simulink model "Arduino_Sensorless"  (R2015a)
settings: Solver=ode45  StartTime=0.0  StopTime=10.0  RelTol=1e-3
libraries: dspsigops x12, arduinolib x11, simulink x7

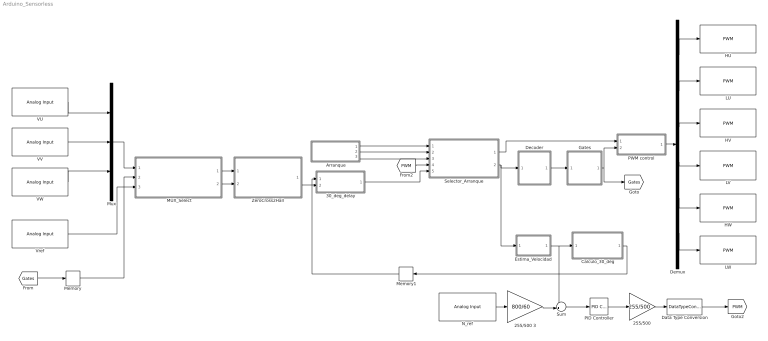
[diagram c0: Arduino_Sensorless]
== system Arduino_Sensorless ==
  " MUX_Select" : Subsystem
  "255/500 " : Gain  Gain=255/500
  255/500 3 : Gain  Gain=800/60
  30_deg_delay : Subsystem
  Arranque : Subsystem
  Calculo_30_deg : Subsystem
  Data Type Conversion : DataTypeConversion  OutDataTypeStr=int16  RndMeth=Round
  Decoder : Subsystem
  Demux : Demux  Outputs=6
  Estima_Velocidad : Subsystem
  Gates : Subsystem
  HU : arduinolib/PWM  pinNumber=3  blockPlatform=arduino
  HV : arduinolib/PWM  pinNumber=6  blockPlatform=arduino
  HW : arduinolib/PWM  pinNumber=10  blockPlatform=arduino
  LU : arduinolib/PWM  pinNumber=5  blockPlatform=arduino
  LV : arduinolib/PWM  pinNumber=9  blockPlatform=arduino
  LW : arduinolib/PWM  pinNumber=11  blockPlatform=arduino
  Memory : Memory
  Memory1 : Memory
  Mux : Mux  Inputs=3
  N_ref : arduinolib/Analog Input  pinNumber=0  sampleTime=1  blockPlatform=arduino
  PID Controller : simulink/Continuous/PID Controller  Controller=PID  TimeDomain=Continuous-time  SampleTime=-1  IntegratorMethod=Forward Euler  FilterMethod=Forward Euler  Form=Parallel  UseFilter=on  ControllerParametersSource=internal  P=500  I=0.1  D=0.08  N=1  InitialConditionSource=internal  InitialConditionForIntegrator=0  InitialConditionForFilter=0  ExternalReset=none  LimitOutput=off  UpperSaturationLimit=inf  LowerSaturationLimit=-inf  LinearizeAsGain=on  AntiWindupMode=none  Kb=1  TrackingMode=off  Kt=1  PParamMin=[]  PParamMax=[]  IParamMin=[]  IParamMax=[]  DParamMin=[]  DParamMax=[]  NParamMin=[]  NParamMax=[]  KbParamMin=[]  KbParamMax=[]  KtParamMin=[]  KtParamMax=[]  POutMin=[]  POutMax=[]  IOutMin=[]  IOutMax=[]  DOutMin=[]  DOutMax=[]  NOutMin=[]  NOutMax=[]  KbOutMin=[]  KbOutMax=[]  KtOutMin=[]  KtOutMax=[]  IntegratorOutMin=[]  IntegratorOutMax=[]  FilterOutMin=[]  FilterOutMax=[]  SumOutMin=[]  SumOutMax=[]  SumI1OutMin=[]  SumI1OutMax=[]  SumI2OutMin=[]  SumI2OutMax=[]  SumI3OutMin=[]  SumI3OutMax=[]  SumDOutMin=[]  SumDOutMax=[]  SaturationOutMin=[]  SaturationOutMax=[]  IntegratorContinuousStateAttributes=''  IntegratorStateMustResolveToSignalObject=off  IntegratorRTWStateStorageClass=Auto  FilterContinuousStateAttributes=''  FilterStateMustResolveToSignalObject=off  FilterRTWStateStorageClass=Auto  DifferentiatorICPrevScaledInput=0  DifferentiatorOutMin=[]  DifferentiatorOutMax=[]
  PWM control : Subsystem
  Selector_Arranque : Subsystem
  Sum : Sum  Inputs=-+|
  VU : arduinolib/Analog Input  pinNumber=1  sampleTime=1  blockPlatform=arduino
  VV : arduinolib/Analog Input  pinNumber=2  sampleTime=1  blockPlatform=arduino
  VW : arduinolib/Analog Input  pinNumber=3  sampleTime=1  blockPlatform=arduino
  Vref : arduinolib/Analog Input  pinNumber=4  sampleTime=1  blockPlatform=arduino
  ZeroCross2Hall : Subsystem
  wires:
  VV/1 -> Mux/2
  VU/1 -> Mux/1
  VW/1 -> Mux/3
  Gates/1(Gates) -> [Gates], PWM control/2(Gates)
  Decoder/1(emf_abc) -> Gates/1("emf_abc ")
  PWM control/1(Pulsos) -> Demux/1
  Demux/1 -> HU/1
  Demux/2 -> LU/1
  Demux/3 -> HV/1
  Demux/4 -> LV/1
  Demux/5 -> HW/1
  Demux/6 -> LW/1
  [Gates] -> Memory/1
  Memory/1 -> " MUX_Select"/2(Gates)
  Mux/1 -> " MUX_Select"/1(Lectura_Fases)
  " MUX_Select"/1(Zero_Crossing) -> ZeroCross2Hall/1(zero_crossing)
  " MUX_Select"/2(Trigger) -> ZeroCross2Hall/2(trigger)
  ZeroCross2Hall/1(Hall) -> 30_deg_delay/2(Hall)
  [PWM] -> Selector_Arranque/4(PWM_Regulacion)
  Arranque/3(Hall_Arranque) -> Selector_Arranque/3(Hal_Arranque)
  Arranque/2(PWM_Arranque) -> Selector_Arranque/2(PWM_Arranque)
  Arranque/1(Trigger) -> Selector_Arranque/1(Trigger)
  Selector_Arranque/2(Hall) -> Estima_Velocidad/1(Hall), Decoder/1("Hall ")
  Selector_Arranque/1(PWM) -> PWM control/1(V control)
  30_deg_delay/1(Hall_Delay) -> Selector_Arranque/5(Hall_Regulacion)
  Vref/1 -> " MUX_Select"/3("V_REF ")
  Sum/1 -> PID Controller/1
  PID Controller/1 -> "255/500 "/1
  "255/500 "/1 -> Data Type Conversion/1
  Data Type Conversion/1 -> [PWM]
  Estima_Velocidad/1(N_est) -> Sum/1, Calculo_30_deg/1(N_rad_s)
  N_ref/1 -> 255/500 3/1
  255/500 3/1 -> Sum/2
  Memory1/1 -> 30_deg_delay/1(30_deg)
  Calculo_30_deg/1(Delay) -> Memory1/1

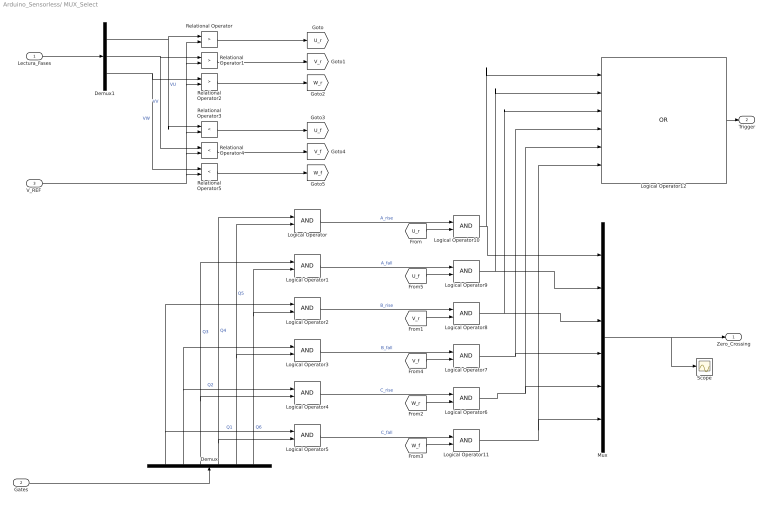
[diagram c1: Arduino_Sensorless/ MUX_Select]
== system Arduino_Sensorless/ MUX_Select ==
  Lectura_Fases : Inport
  Gates : Inport  Port=2
  "V_REF " : Inport  Port=3
  Demux : Demux  Outputs=6
  Demux1 : Demux  Outputs=3
  Logical Operator{,1..11} (12 alike) : Logic  IconShape=distinctive  AllPortsSameDT=off  OutDataTypeStr=boolean
  Logical Operator12 : Logic  Operator=OR  Inputs=6  AllPortsSameDT=off  OutDataTypeStr=boolean
  Mux : Mux  Inputs=6
  Relational Operator : RelationalOperator  Operator=>  OutDataTypeStr=boolean
  Relational Operator1 : RelationalOperator  Operator=>  OutDataTypeStr=boolean
  Relational Operator2 : RelationalOperator  Operator=>  OutDataTypeStr=boolean
  Relational Operator3 : RelationalOperator  Operator=<  OutDataTypeStr=boolean
  Relational Operator4 : RelationalOperator  Operator=<  OutDataTypeStr=boolean
  Relational Operator5 : RelationalOperator  Operator=<  OutDataTypeStr=boolean
  Scope : Scope
  Zero_Crossing : Outport
  Trigger : Outport  Port=2
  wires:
  Gates/1 -> Demux/1
  Demux/1 -> Logical Operator5/1, Logical Operator2/1  "Q1"
  Demux/2 -> Logical Operator4/1, Logical Operator3/1  "Q2"
  Demux/3 -> Logical Operator4/2, Logical Operator1/1  "Q3"
  Demux/4 -> Logical Operator5/2, Logical Operator/1  "Q4"
  Demux/5 -> Logical Operator3/2, Logical Operator/2  "Q5"
  Demux/6 -> Logical Operator2/2, Logical Operator1/2  "Q6"
  Logical Operator2/1 -> Logical Operator8/1  "B_rise"
  Logical Operator3/1 -> Logical Operator7/1  "B_fall"
  Logical Operator/1 -> Logical Operator10/1  "A_rise"
  Logical Operator1/1 -> Logical Operator9/1  "A_fall"
  Logical Operator4/1 -> Logical Operator6/1  "C_rise"
  Logical Operator5/1 -> Logical Operator11/1  "C_fall"
  Relational Operator3/1 -> [U_f]
  Relational Operator4/1 -> [V_f]
  Relational Operator5/1 -> [W_f]
  [U_r] -> Logical Operator10/2
  [U_f] -> Logical Operator9/2
  [V_r] -> Logical Operator8/2
  [V_f] -> Logical Operator7/2
  [W_r] -> Logical Operator6/2
  [W_f] -> Logical Operator11/2
  Mux/1 -> Scope/1, Zero_Crossing/1
  Logical Operator6/1 -> Logical Operator12/5, Mux/5
  Logical Operator11/1 -> Mux/6, Logical Operator12/6
  Logical Operator7/1 -> Logical Operator12/4, Mux/4
  Logical Operator8/1 -> Logical Operator12/3, Mux/3
  Logical Operator9/1 -> Logical Operator12/2, Mux/2
  Logical Operator10/1 -> Logical Operator12/1, Mux/1
  Logical Operator12/1 -> Trigger/1
  Lectura_Fases/1 -> Demux1/1
  "V_REF "/1 -> Relational Operator4/2, Relational Operator3/2, Relational Operator2/2, Relational Operator1/2, Relational Operator/2, Relational Operator5/2
  Demux1/3 -> Relational Operator5/1, Relational Operator2/1  "VW"
  Demux1/1 -> Relational Operator3/1, Relational Operator/1  "VU"
  Demux1/2 -> Relational Operator4/1, Relational Operator1/1  "VV"
  Relational Operator2/1 -> [W_r]
  Relational Operator1/1 -> [V_r]
  Relational Operator/1 -> [U_r]

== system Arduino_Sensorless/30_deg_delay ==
  30_deg : Inport
  Hall : Inport  Port=2
  Data Type Conversion : DataTypeConversion  OutDataTypeStr=double
  Data Type Conversion1 : DataTypeConversion  OutDataTypeStr=boolean
  Variable Time Delay : VariableTransportDelay  MaximumDelay=10  MaximumPoints=256  FixedBuffer=on
  Hall_Delay : Outport
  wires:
  Hall/1 -> Data Type Conversion/1
  Data Type Conversion/1 -> Variable Time Delay/1
  30_deg/1 -> Variable Time Delay/2
  Variable Time Delay/1 -> Data Type Conversion1/1
  Data Type Conversion1/1 -> Hall_Delay/1

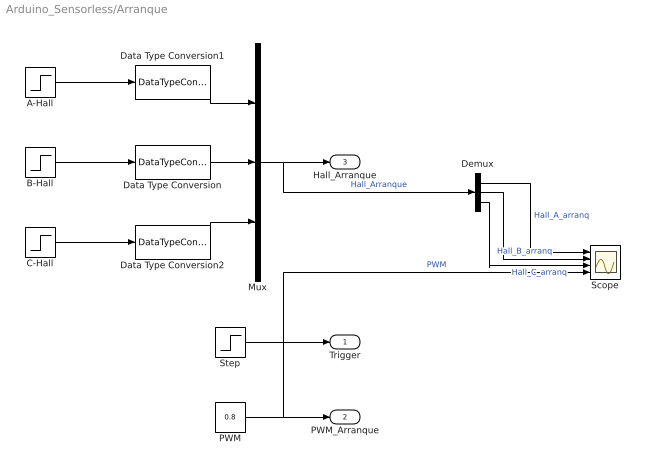
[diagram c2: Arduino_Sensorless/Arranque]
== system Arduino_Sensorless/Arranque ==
  A-Hall : Step  Time=8.364E-3  Before=1  After=0  SampleTime=0
  B-Hall : Step  Time=5.8145E-3  SampleTime=0
  C-Hall : Step  Time=10.8E-3  SampleTime=0
  Data Type Conversion : DataTypeConversion  OutDataTypeStr=boolean
  Data Type Conversion1 : DataTypeConversion  OutDataTypeStr=boolean
  Data Type Conversion2 : DataTypeConversion  OutDataTypeStr=boolean
  Demux : Demux  Outputs=3
  Mux : Mux  Inputs=3
  PWM : Constant  Value=0.8
  Scope : Scope  NumInputPorts=4
  Step : Step  Time=13.25E-3  Before=0.5  After=-0.5  SampleTime=0
  Trigger : Outport
  PWM_Arranque : Outport  Port=2
  Hall_Arranque : Outport  Port=3
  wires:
  B-Hall/1 -> Data Type Conversion/1
  C-Hall/1 -> Data Type Conversion2/1
  A-Hall/1 -> Data Type Conversion1/1
  Data Type Conversion/1 -> Mux/2
  Data Type Conversion1/1 -> Mux/1
  Data Type Conversion2/1 -> Mux/3
  Mux/1 -> Demux/1, Hall_Arranque/1  "Hall_Arranque"
  Step/1 -> Trigger/1
  PWM/1 -> Scope/4, PWM_Arranque/1  "PWM"
  Demux/1 -> Scope/1  "Hall_A_arranq"
  Demux/2 -> Scope/2  "Hall_B_arranq"
  Demux/3 -> Scope/3  "Hall_C_arranq"

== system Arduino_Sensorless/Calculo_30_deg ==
  N_rad_s : Inport
  30_deg : Constant  Value=1/12
  Divide : Product  Inputs=*/
  Saturation : Saturate  UpperLimit=inf  LowerLimit=10
  Scope : Scope
  Delay : Outport
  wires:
  30_deg/1 -> Divide/1
  Divide/1 -> Scope/1, Delay/1
  N_rad_s/1 -> Saturation/1
  Saturation/1 -> Divide/2

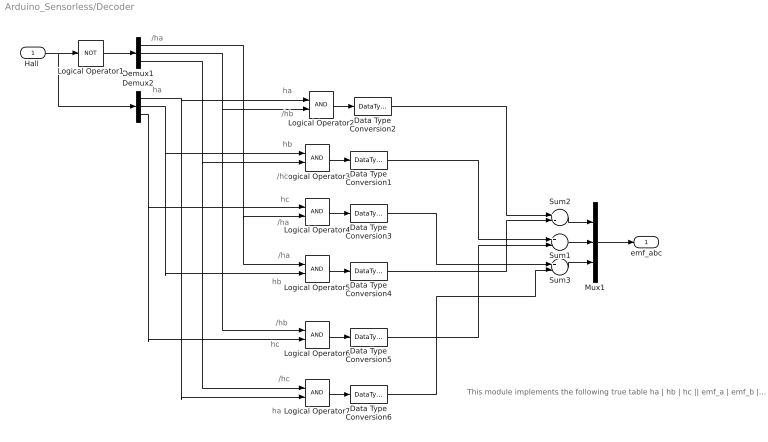
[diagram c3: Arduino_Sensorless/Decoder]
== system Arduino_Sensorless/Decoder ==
  note: /ha
  note: ha
  note: ha
  note: /hb
  note: hb
  note: /hc
  note: hc
  note: /ha
  note: /ha
  note: hb
  note: /hb
  note: hc
  note: /hc
  note: ha
  note: This module implements the following true table ha | hb | hc || emf_a | emf_b | emf_c -------------------------------------------------------------------------------- 0 0 0 0 0 0 0 0 1 0 -1 +1 0 1 0 -1 +1 0 0 1 1 -1 0 +1 1 0 0 +1 0 -1 1 0 1 +1 -1 0 1 1 0 0 +1 -1 1 1 1 0 0 0
  "Hall " : Inport
  Data Type Conversion{1..6} (6 alike) : DataTypeConversion
  Demux1 : Demux  Outputs=3
  Demux2 : Demux  Outputs=3
  Logical Operator1 : Logic  Operator=NOT  AllPortsSameDT=off  OutDataTypeStr=boolean
  Logical Operator{2..7} (6 alike) : Logic  AllPortsSameDT=off  OutDataTypeStr=boolean
  Mux1 : Mux  Inputs=3
  Sum1 : Sum  Inputs=+-  OutDataTypeStr=double
  Sum2 : Sum  Inputs=+-  OutDataTypeStr=double
  Sum3 : Sum  Inputs=+-  OutDataTypeStr=double
  emf_abc : Outport
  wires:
  "Hall "/1 -> Logical Operator1/1, Demux2/1
  Logical Operator1/1 -> Demux1/1
  Demux2/3 -> Logical Operator4/1, Logical Operator6/2
  Demux2/2 -> Logical Operator3/1, Logical Operator5/2
  Demux2/1 -> Logical Operator2/1, Logical Operator7/2
  Demux1/3 -> Logical Operator3/2, Logical Operator7/1
  Demux1/2 -> Logical Operator2/2, Logical Operator6/1
  Demux1/1 -> Logical Operator4/2, Logical Operator5/1
  Logical Operator2/1 -> Data Type Conversion2/1
  Sum2/1 -> Mux1/1
  Sum1/1 -> Mux1/2
  Sum3/1 -> Mux1/3
  Mux1/1 -> emf_abc/1
  Logical Operator3/1 -> Data Type Conversion1/1
  Logical Operator4/1 -> Data Type Conversion3/1
  Logical Operator5/1 -> Data Type Conversion4/1
  Logical Operator6/1 -> Data Type Conversion5/1
  Logical Operator7/1 -> Data Type Conversion6/1
  Data Type Conversion2/1 -> Sum2/1
  Data Type Conversion4/1 -> Sum2/2
  Data Type Conversion1/1 -> Sum1/1
  Data Type Conversion5/1 -> Sum1/2
  Data Type Conversion3/1 -> Sum3/1
  Data Type Conversion6/1 -> Sum3/2

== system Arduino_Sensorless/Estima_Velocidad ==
  Hall : Inport
  Demux : Demux  Outputs=3
  Estima_v_Fase_A : Subsystem
  Estima_v_Fase_B : Subsystem
  Estima_v_Fase_C : Subsystem
  Seleccion_estimada : Subsystem
  N_est : Outport
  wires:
  Demux/1 -> Estima_v_Fase_A/1(Hall_i)
  Hall/1 -> Seleccion_estimada/4(Hall), Demux/1
  Demux/3 -> Estima_v_Fase_C/1(Hall_i)
  Demux/2 -> Estima_v_Fase_B/1(Hall_i)
  Estima_v_Fase_A/1(Estimada_i) -> Seleccion_estimada/1(Estimada_A)
  Estima_v_Fase_B/1(Estimada_i) -> Seleccion_estimada/2(Estimada_B)
  Estima_v_Fase_C/1(Estimada_i) -> Seleccion_estimada/3(Estimada_C)
  Seleccion_estimada/1(Out1) -> N_est/1

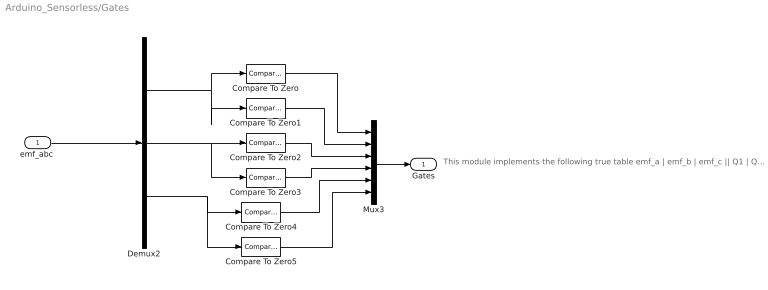
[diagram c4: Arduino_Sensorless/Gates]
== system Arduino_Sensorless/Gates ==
  note: This module implements the following true table emf_a | emf_b | emf_c || Q1 | Q2 | Q3 | Q4 | Q5 | Q6 ------------------------------------------------------------------------------------------------------------------ 0 0 0 0 0 0 0 0 0 0 -1 +1 0 0 0 1 1 0 -1 +1 0 0 1 1 0 0 0 -1 0 +1 0 1 0 0 1 0 +1 0 -1 1 0 0 0 0 1 +1 -1 0 1 0 0 1 0 0 0 +1 -1 0 0 1 0 0 1 0 0 0 0 0 0 0 0 0
  "emf_abc " : Inport
  Compare To Zero : simulink/Logic and Bit Operations/Compare To Zero  relop=>  OutDataTypeStr=boolean  ZeroCross=off
  Compare To Zero1 : simulink/Logic and Bit Operations/Compare To Zero  relop=<  OutDataTypeStr=boolean  ZeroCross=off
  Compare To Zero2 : simulink/Logic and Bit Operations/Compare To Zero  relop=>  OutDataTypeStr=boolean  ZeroCross=off
  Compare To Zero3 : simulink/Logic and Bit Operations/Compare To Zero  relop=<  OutDataTypeStr=boolean  ZeroCross=off
  Compare To Zero4 : simulink/Logic and Bit Operations/Compare To Zero  relop=>  OutDataTypeStr=boolean  ZeroCross=off
  Compare To Zero5 : simulink/Logic and Bit Operations/Compare To Zero  relop=<  OutDataTypeStr=boolean  ZeroCross=off
  Demux2 : Demux  Outputs=3
  Mux3 : Mux  Inputs=6
  Gates : Outport
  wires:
  "emf_abc "/1 -> Demux2/1
  Mux3/1 -> Gates/1
  Demux2/1 -> Compare To Zero/1, Compare To Zero1/1
  Demux2/2 -> Compare To Zero2/1, Compare To Zero3/1
  Demux2/3 -> Compare To Zero4/1, Compare To Zero5/1
  Compare To Zero/1 -> Mux3/1
  Compare To Zero1/1 -> Mux3/2
  Compare To Zero2/1 -> Mux3/3
  Compare To Zero3/1 -> Mux3/4
  Compare To Zero4/1 -> Mux3/5
  Compare To Zero5/1 -> Mux3/6

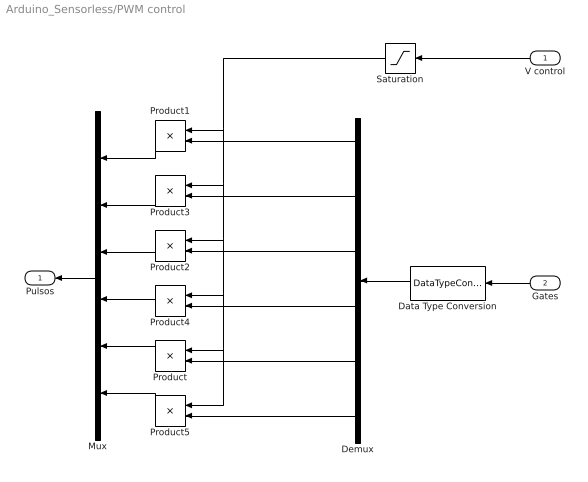
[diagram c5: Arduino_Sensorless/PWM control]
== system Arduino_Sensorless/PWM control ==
  V control : Inport
  Gates : Inport  Port=2
  Data Type Conversion : DataTypeConversion  OutDataTypeStr=double
  Demux : Demux  Outputs=6
  Mux : Mux  Inputs=6
  Product{,1..5} (6 alike) : Product
  Saturation : Saturate  UpperLimit=255  LowerLimit=0
  Pulsos : Outport
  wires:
  Gates/1 -> Data Type Conversion/1
  Data Type Conversion/1 -> Demux/1
  Mux/1 -> Pulsos/1
  Product1/1 -> Mux/1
  Product2/1 -> Mux/3
  Product/1 -> Mux/5
  Demux/5 -> Product/2
  Demux/3 -> Product2/2
  Demux/1 -> Product1/2
  V control/1 -> Saturation/1
  Product5/1 -> Mux/6
  Demux/6 -> Product5/2
  Product4/1 -> Mux/4
  Demux/4 -> Product4/2
  Product3/1 -> Mux/2
  Demux/2 -> Product3/2
  Saturation/1 -> Product3/1, Product4/1, Product/1, Product5/1, Product2/1, Product1/1

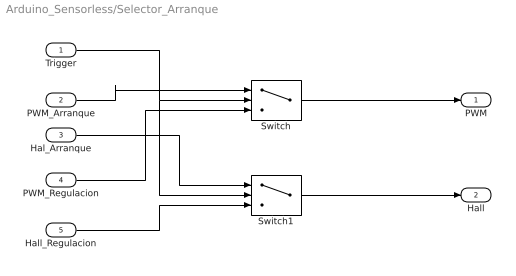
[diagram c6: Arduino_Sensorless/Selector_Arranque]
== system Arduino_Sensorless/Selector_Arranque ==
  Trigger : Inport
  PWM_Arranque : Inport  Port=2
  Hal_Arranque : Inport  Port=3
  PWM_Regulacion : Inport  Port=4
  Hall_Regulacion : Inport  Port=5
  Switch : Switch  Criteria=u2 > Threshold
  Switch1 : Switch  Criteria=u2 > Threshold
  PWM : Outport
  Hall : Outport  Port=2
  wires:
  Trigger/1 -> Switch1/2, Switch/2
  Hall_Regulacion/1 -> Switch1/3
  PWM_Regulacion/1 -> Switch/3
  Hal_Arranque/1 -> Switch1/1
  PWM_Arranque/1 -> Switch/1
  Switch/1 -> PWM/1
  Switch1/1 -> Hall/1

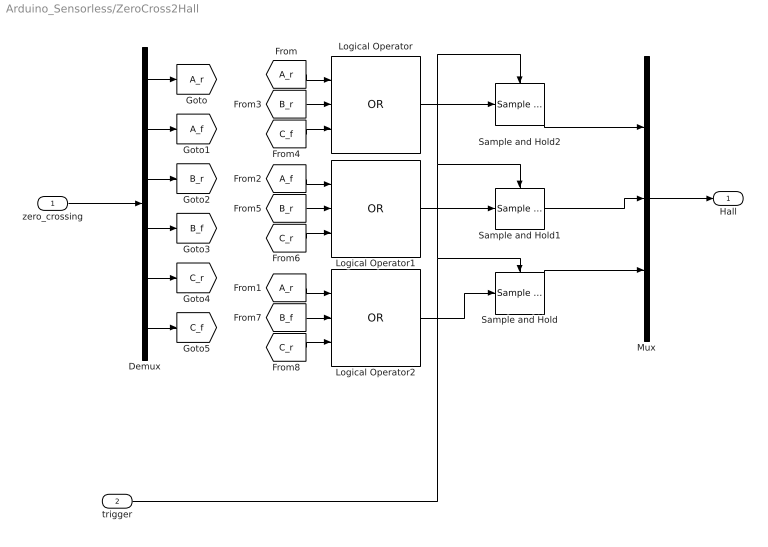
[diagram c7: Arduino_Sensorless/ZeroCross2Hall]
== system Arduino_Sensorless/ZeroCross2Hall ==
  zero_crossing : Inport
  trigger : Inport  Port=2
  Demux : Demux  Outputs=6
  Logical Operator : Logic  Operator=OR  Inputs=3  IconShape=distinctive  AllPortsSameDT=off  OutDataTypeStr=boolean
  Logical Operator1 : Logic  Operator=OR  Inputs=3  IconShape=distinctive  AllPortsSameDT=off  OutDataTypeStr=boolean
  Logical Operator2 : Logic  Operator=OR  Inputs=3  IconShape=distinctive  AllPortsSameDT=off  OutDataTypeStr=boolean
  Mux : Mux  Inputs=3
  Sample and Hold : dspsigops/Sample and Hold  trig=Rising edge  initCond=0  latchinput=off
  Sample and Hold1 : dspsigops/Sample and Hold  trig=Rising edge  initCond=0  latchinput=off
  Sample and Hold2 : dspsigops/Sample and Hold  trig=Rising edge  initCond=0  latchinput=off
  Hall : Outport
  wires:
  zero_crossing/1 -> Demux/1
  Mux/1 -> Hall/1
  trigger/1 -> Sample and Hold/Trigger, Sample and Hold1/Trigger, Sample and Hold2/Trigger
  Logical Operator2/1 -> Sample and Hold/1
  Sample and Hold/1 -> Mux/3
  Sample and Hold1/1 -> Mux/2
  Sample and Hold2/1 -> Mux/1
  Logical Operator1/1 -> Sample and Hold1/1
  Logical Operator/1 -> Sample and Hold2/1
  Demux/1 -> [A_r]
  Demux/6 -> [C_f]
  Demux/3 -> [B_r]
  Demux/2 -> [A_f]
  Demux/4 -> [B_f]
  Demux/5 -> [C_r]
  [A_r] -> Logical Operator2/1
  [A_r] -> Logical Operator/1
  [A_f] -> Logical Operator1/1
  [B_r] -> Logical Operator/2
  [C_f] -> Logical Operator/3
  [B_r] -> Logical Operator1/2
  [C_r] -> Logical Operator1/3
  [C_r] -> Logical Operator2/3
  [B_f] -> Logical Operator2/2

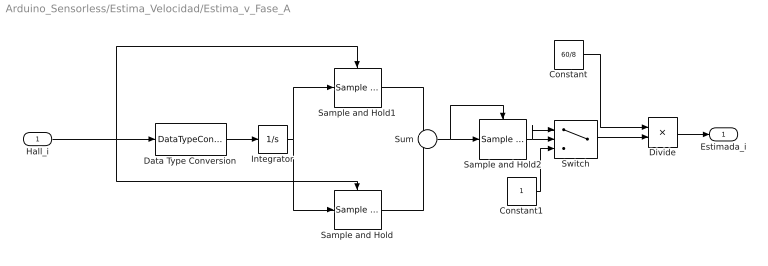
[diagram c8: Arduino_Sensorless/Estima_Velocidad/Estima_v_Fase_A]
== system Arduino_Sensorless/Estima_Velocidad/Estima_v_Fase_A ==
  Hall_i : Inport
  Constant : Constant  Value=60/8
  Constant1 : Constant
  Data Type Conversion : DataTypeConversion  OutDataTypeStr=double
  Divide : Product  Inputs=*/
  Integrator : Integrator
  Sample and Hold : dspsigops/Sample and Hold  trig=Rising edge  initCond=0  latchinput=off
  Sample and Hold1 : dspsigops/Sample and Hold  trig=Falling edge  initCond=0  latchinput=off
  Sample and Hold2 : dspsigops/Sample and Hold  trig=Rising edge  initCond=0  latchinput=off
  Sum : Sum  Inputs=+|-
  Switch : Switch  Criteria=u2 > Threshold
  Estimada_i : Outport
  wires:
  Hall_i/1 -> Data Type Conversion/1, Sample and Hold/Trigger, Sample and Hold1/Trigger
  Integrator/1 -> Sample and Hold1/1, Sample and Hold/1
  Sample and Hold/1 -> Sum/2
  Sample and Hold1/1 -> Sum/1
  Sum/1 -> Sample and Hold2/Trigger, Sample and Hold2/1
  Sample and Hold2/1 -> Switch/1, Switch/2
  Constant/1 -> Divide/1
  Switch/1 -> Divide/2
  Constant1/1 -> Switch/3
  Divide/1 -> Estimada_i/1
  Data Type Conversion/1 -> Integrator/1

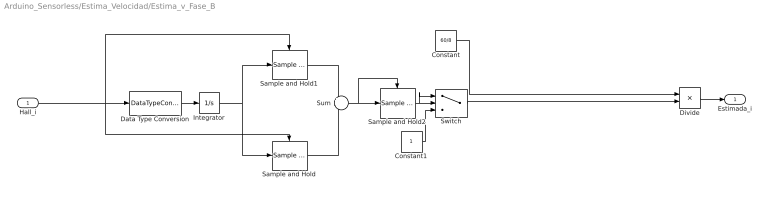
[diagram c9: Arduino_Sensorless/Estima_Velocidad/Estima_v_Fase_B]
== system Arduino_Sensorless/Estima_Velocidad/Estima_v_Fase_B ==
  Hall_i : Inport
  Constant : Constant  Value=60/8
  Constant1 : Constant
  Data Type Conversion : DataTypeConversion  OutDataTypeStr=double
  Divide : Product  Inputs=*/
  Integrator : Integrator
  Sample and Hold : dspsigops/Sample and Hold  trig=Rising edge  initCond=0  latchinput=off
  Sample and Hold1 : dspsigops/Sample and Hold  trig=Falling edge  initCond=0  latchinput=off
  Sample and Hold2 : dspsigops/Sample and Hold  trig=Rising edge  initCond=0  latchinput=off
  Sum : Sum  Inputs=+|-
  Switch : Switch  Criteria=u2 > Threshold
  Estimada_i : Outport
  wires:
  Hall_i/1 -> Data Type Conversion/1, Sample and Hold/Trigger, Sample and Hold1/Trigger
  Integrator/1 -> Sample and Hold1/1, Sample and Hold/1
  Sample and Hold/1 -> Sum/2
  Sample and Hold1/1 -> Sum/1
  Sum/1 -> Sample and Hold2/Trigger, Sample and Hold2/1
  Sample and Hold2/1 -> Switch/1, Switch/2
  Constant/1 -> Divide/1
  Switch/1 -> Divide/2
  Constant1/1 -> Switch/3
  Divide/1 -> Estimada_i/1
  Data Type Conversion/1 -> Integrator/1

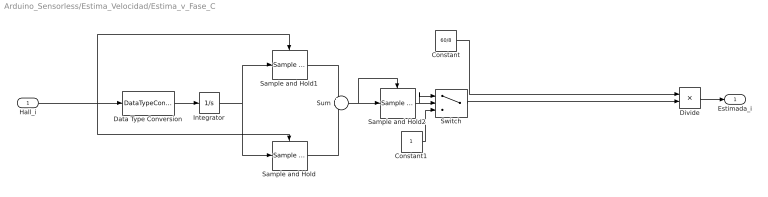
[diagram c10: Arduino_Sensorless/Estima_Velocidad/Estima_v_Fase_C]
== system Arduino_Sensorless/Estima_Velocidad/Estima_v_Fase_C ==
  Hall_i : Inport
  Constant : Constant  Value=60/8
  Constant1 : Constant
  Data Type Conversion : DataTypeConversion  OutDataTypeStr=double
  Divide : Product  Inputs=*/
  Integrator : Integrator
  Sample and Hold : dspsigops/Sample and Hold  trig=Rising edge  initCond=0  latchinput=off
  Sample and Hold1 : dspsigops/Sample and Hold  trig=Falling edge  initCond=0  latchinput=off
  Sample and Hold2 : dspsigops/Sample and Hold  trig=Rising edge  initCond=0  latchinput=off
  Sum : Sum  Inputs=+|-
  Switch : Switch  Criteria=u2 > Threshold  Threshold=3E-5
  Estimada_i : Outport
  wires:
  Hall_i/1 -> Data Type Conversion/1, Sample and Hold/Trigger, Sample and Hold1/Trigger
  Integrator/1 -> Sample and Hold1/1, Sample and Hold/1
  Sample and Hold/1 -> Sum/2
  Sample and Hold1/1 -> Sum/1
  Sum/1 -> Sample and Hold2/Trigger, Sample and Hold2/1
  Sample and Hold2/1 -> Switch/1, Switch/2
  Constant/1 -> Divide/1
  Switch/1 -> Divide/2
  Constant1/1 -> Switch/3
  Divide/1 -> Estimada_i/1
  Data Type Conversion/1 -> Integrator/1

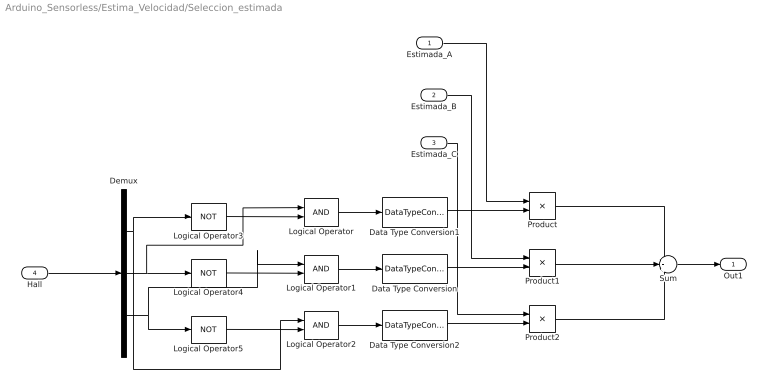
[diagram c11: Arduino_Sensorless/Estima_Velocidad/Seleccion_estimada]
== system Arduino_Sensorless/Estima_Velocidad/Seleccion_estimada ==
  Estimada_A : Inport
  Estimada_B : Inport  Port=2
  Estimada_C : Inport  Port=3
  Hall : Inport  Port=4
  Data Type Conversion : DataTypeConversion  OutDataTypeStr=double
  Data Type Conversion1 : DataTypeConversion  OutDataTypeStr=double
  Data Type Conversion2 : DataTypeConversion  OutDataTypeStr=double
  Demux : Demux  Outputs=3
  Logical Operator : Logic  IconShape=distinctive  AllPortsSameDT=off  OutDataTypeStr=boolean
  Logical Operator1 : Logic  IconShape=distinctive  AllPortsSameDT=off  OutDataTypeStr=boolean
  Logical Operator2 : Logic  IconShape=distinctive  AllPortsSameDT=off  OutDataTypeStr=boolean
  Logical Operator3 : Logic  Operator=NOT  IconShape=distinctive  AllPortsSameDT=off  OutDataTypeStr=boolean
  Logical Operator4 : Logic  Operator=NOT  IconShape=distinctive  AllPortsSameDT=off  OutDataTypeStr=boolean
  Logical Operator5 : Logic  Operator=NOT  IconShape=distinctive  AllPortsSameDT=off  OutDataTypeStr=boolean
  Product : Product
  Product1 : Product
  Product2 : Product
  Sum : Sum  Inputs=+++
  Out1 : Outport
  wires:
  Hall/1 -> Demux/1
  Product/1 -> Sum/1
  Product1/1 -> Sum/2
  Product2/1 -> Sum/3
  Logical Operator3/1 -> Logical Operator/2
  Logical Operator4/1 -> Logical Operator1/2
  Logical Operator5/1 -> Logical Operator2/2
  Demux/3 -> Logical Operator1/1, Logical Operator5/1
  Demux/2 -> Logical Operator/1, Logical Operator4/1
  Demux/1 -> Logical Operator2/1, Logical Operator3/1
  Logical Operator1/1 -> Data Type Conversion/1
  Logical Operator2/1 -> Data Type Conversion2/1
  Logical Operator/1 -> Data Type Conversion1/1
  Sum/1 -> Out1/1
  Estimada_C/1 -> Product2/1
  Data Type Conversion2/1 -> Product2/2
  Data Type Conversion/1 -> Product1/2
  Data Type Conversion1/1 -> Product/2
  Estimada_B/1 -> Product1/1
  Estimada_A/1 -> Product/1
